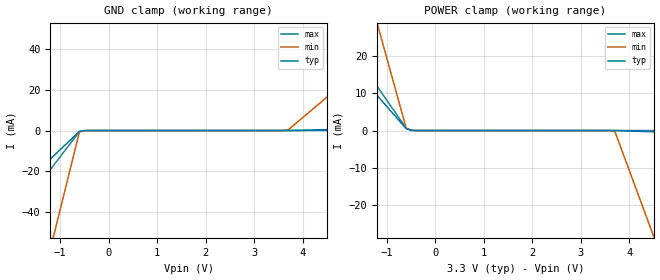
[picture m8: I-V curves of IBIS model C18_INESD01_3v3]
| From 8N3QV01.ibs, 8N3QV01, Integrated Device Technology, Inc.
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[Model] C18_INESD01_3v3
Model_type   Input
Polarity   Non-Inverting
Vinl = 0.8V
Vinh = 2.0V
|   typ   min   max
C_comp   2pF   1.5pF   2.5pF
|   typ   min   max
[Voltage range]   3.3V   3.135V   3.465V
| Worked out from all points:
|   GND clamp passes 1 mA (typ) near -0.62 V on its own axis
|   POWER clamp passes 1 mA (typ) near -0.63 V on its own axis
[GND_clamp]
|Voltage   I (typ)   I (min)   I (max)
-3.3V     -61.26mA   -259.6mA   -84.33mA
-2.9V     -52.25mA   -221.2mA   -71.91mA
-2.8V     -49.99mA   -211.6mA   -68.81mA
-2.3V     -38.73mA   -163.7mA   -53.29mA
-2.2V     -36.48mA   -154.1mA   -50.18mA
-1.2V     -13.96mA   -58.22mA   -19.14mA
-1.1V     -11.7mA    -48.63mA   -16.04mA
-600mV    -441.3uA   -687.4uA   -515uA
-400mV    -3.107uA   -5.521uA   -1.269uA
3.7V      3.349uA    270.4uA    1.215nA
6.2V      1.303mA    50.31mA    2.8uA
6.6V      1.511mA    58.32mA    3.248uA
[Power_clamp]
|Voltage   I (typ)   I (min)   I (max)
-3.3V     40.6mA     127.8mA    51.18mA
-2.5V     28.72mA    90.08mA    36.19mA
-2.4V     27.23mA    85.36mA    34.32mA
-2.1V     22.78mA    71.23mA    28.7mA
-2V       21.29mA    66.52mA    26.83mA
-1.2V     9.404mA    28.83mA    11.84mA
-1.1V     7.918mA    24.12mA    9.964mA
-600mV    489.9uA    564uA      596.7uA
-500mV    55.35uA    63.4uA     49.99uA
3.7V      -3.107uA   -289uA     -1.615nA
4.5V      -343.9uA   -28.48mA   -808.2nA
6.6V      -1.239mA   -102.5mA   -2.926uA
